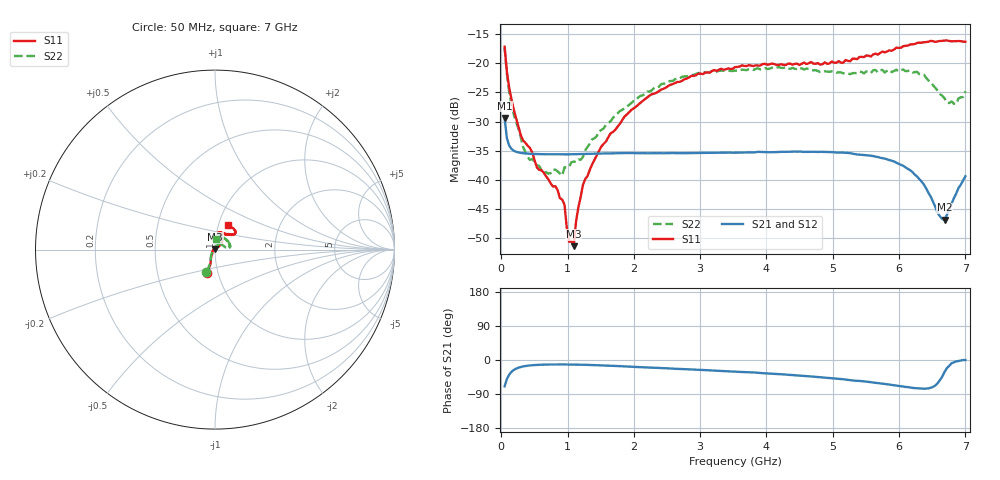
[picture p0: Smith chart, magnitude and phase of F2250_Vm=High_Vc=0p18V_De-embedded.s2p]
! Integrated Device Technology
! Corporate Headquarters
! 6024 Silver Creek Valley Road
! San Jose, CA 95138  USA
! Phone:  1-408-284-8200
! Toll Free:  1-800-223-1366
! Webpage:  http://www.idt.com/
! Timing and RF Division
! 515 Groton Road, Suite 102
! Westford, MA 01886-6024
! Device:  F2250
! Description: Voltage Variable RF Attenuator
! Frequency:  50.0 -  6000.00 MHz
! Package:  3x3 mm Thin QFN Plastic Package: 16 pin
! Ports:  2 RF, 3 DC
!  Pin  1  = GND
!  Pin  2  = NC
!  Pin  3  = RF1  = Port 1
!  Pin  4  = NC
!  Pin  5  = GND
!  Pin  6  = GND
!  Pin  7  = GND
!  Pin  8  = GND
!  Pin  9  = NC
!  Pin 10  = RF2  = Port 2
!  Pin 11  = NC
!  Pin 12  = GND
!  Pin 13  = GND
!  Pin 14  = VCNTRL
!  Pin 15  = VDD
!  Pin 16  = VMODE
! Vcntrl:  0.180 Volts
! Vmode:  +3.300 Volts
! Vdd:  +3.30  Volts
! Current:  1.243 mA
! Data:  The device was measured on a the F2250 evaluation board which has
!  individual transmission lines to the RF pins.  Data was collected
!  using a calibrated network analyzer.  The evaluation board was
!  de-embedded using a TRL calibration technique.
!  The reference plane is the edge of the package pin.
! Misc:  SN 10
!  Action Tracker AT0258
! Date Measured:  2014-11-26
! Date:  2015-10-15  MJV
! Note:
!  Integrated Device Technology supplies this data as a sample of measured
!  data at the package pin for this product.  Your particular data for this
!  product may vary.
!  Data was taken at 25 degrees C.
!  Integrated Device Technology reserves the right to change this data at anytime.
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# GHz S dB R 50
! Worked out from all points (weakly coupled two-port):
!   201 points, 50 MHz to 7 GHz, reference 50 ohm
!   highest |S21| = -29.38 dB at 50 MHz (marker M1); lowest = -46.8 dB at 6.687 GHz (marker M2)
!   lowest |S11| = -51.3 dB at 1.093 GHz (marker M3), VSWR 1.01, Z = 50 + j0.272 ohm
!   |S11| at or under -10 dB: start of sweep to end of sweep
!   |S22| runs from -39.2 to -17.4 dB; largest |S21 - S12| = 6.1e-05
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0.05  -17.18 -108.5  -29.38 -69.5  -29.38 -69.5  -17.37 -110.6
0.08475  -21.47 -107.4  -32.86 -50.1  -32.86 -50.1  -21.87 -109.0
0.15425  -26.23 -116.6  -34.68 -31.0  -34.68 -31.0  -27.10 -120.7
0.29325  -32.28 -127.5  -35.35 -18.5  -35.35 -18.4  -32.68 -133.6
0.3975  -34.12 -142.2  -35.48 -15.0  -35.48 -15.0  -36.08 -158.4
0.5365  -37.84 -154.5  -35.55 -12.9  -35.55 -12.9  -37.48 180.0
0.64075  -38.75 -162.5  -35.58 -12.2  -35.58 -12.2  -38.89 160.7
0.91875  -43.34 156.0  -35.60 -11.8  -35.60 -11.8  -39.22 127.9
0.9535  -44.22 171.0  -35.60 -11.8  -35.60 -11.8  -37.81 124.2
1.023  -50.59 140.2  -35.59 -11.9  -35.59 -11.9  -37.74 108.1
1.0925  -51.32 89.5  -35.57 -12.0  -35.57 -12.0  -36.84 98.7
1.12725  -47.12 61.9  -35.56 -12.1  -35.56 -12.1  -36.92 91.7
1.2315  -40.83 40.9  -35.52 -12.5  -35.52 -12.5  -36.06 77.3
1.6485  -32.02 41.3  -35.44 -15.2  -35.44 -15.2  -29.92 60.0
2.37825  -24.76 46.7  -35.40 -21.0  -35.40 -21.0  -24.03 53.9
3.525  -20.65 71.7  -35.32 -30.6  -35.32 -30.7  -21.26 72.9
4.7065  -20.06 72.0  -35.15 -43.9  -35.15 -43.9  -21.20 70.4
5.85325  -17.79 40.5  -36.58 -64.8  -36.58 -65.0  -21.13 23.4
6.27025  -16.53 39.4  -39.39 -74.5  -39.40 -74.6  -21.46 8.6
6.68725  -16.11 47.9  -46.80 -31.2  -46.77 -30.7  -26.02 28.5
6.861  -16.22 54.5  -42.31 -3.7  -42.27 -3.7  -26.97 57.4
7  -16.32 62.4  -39.35 -0.1  -39.32 -0.3  -24.81 83.6
